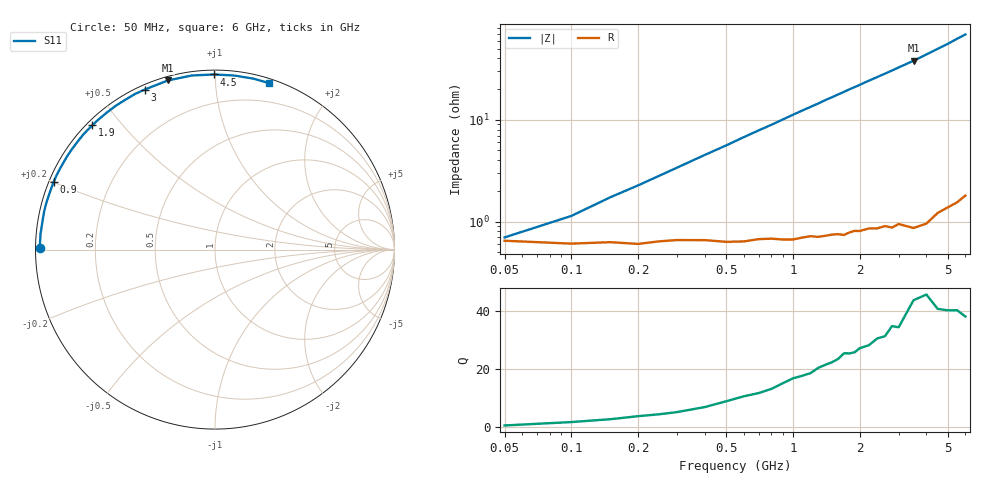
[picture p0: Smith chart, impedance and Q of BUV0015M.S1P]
! Infineon Technologies  Discrete & RF Semiconductors
! BB 833
! Si Tuning Diode in SOD323
! VR =
! S-Parameters:  June  1999
# GHz  S  MA  R  50
!  f  S11
! GHz  MAG  ANG
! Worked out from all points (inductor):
!   34 points, 50 MHz to 6 GHz, reference 50 ohm
!   read as one part to ground: L = 1.75 nH near 200 MHz
!   highest Q = 43.9 at 3.5 GHz (marker M1), where L = 1.73 nH
!   S11 on the Smith chart (normalised r, x): 50 MHz: 0.01, +0.01; 900 MHz: 0.01, +0.20; 1.9 GHz: 0.02, +0.42; 3 GHz: 0.02, +0.65; 4.5 GHz: 0.02, +0.99; 6 GHz: 0.04, +1.38
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0.05  0.9744 179.4
0.1  0.976 177.8
0.15  0.9752 176.3
0.2  0.9762 175.0
0.4  0.9743 169.8
0.5  0.9753 167.3
0.6  0.9752 164.7
0.8  0.974 159.8
0.9  0.9747 157.3
1  0.9749 154.8
1.1  0.9741 152.4
1.3  0.9742 147.8
1.4  0.9739 145.4
1.6  0.9736 141.0
1.7  0.9745 138.8
1.8  0.9734 136.6
1.9  0.9728 134.6
2  0.9733 132.5
2.2  0.9727 128.4
2.4  0.9735 124.6
2.8  0.9749 117.3
3  0.9738 113.7
3.5  0.9783 105.6
4  0.9786 97.6
4.5  0.9758 90.3
5  0.9757 83.8
5.5  0.9762 77.4
6  0.9754 72.0
